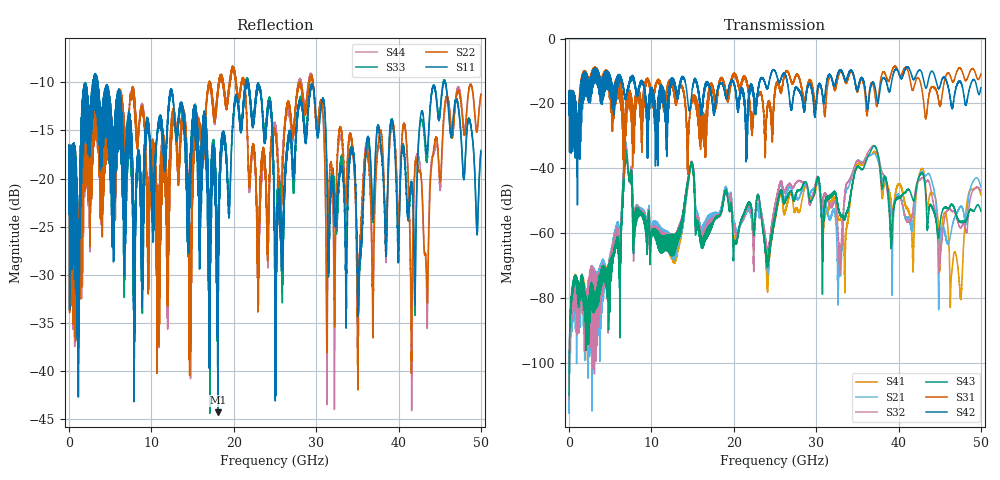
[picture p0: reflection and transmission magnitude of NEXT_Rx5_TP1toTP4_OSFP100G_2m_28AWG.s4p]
! Touchstone data
! Created: 27-Feb-2019 by IdEM 12 (12.1.0)
! COMMENTS
!  Created Wed Feb 27 12:03:36 2019
!  64 Port Network Data from SP1.SP block
!  freq  magS1_1  angS1_1  magS1_2  angS1_2  magS1_3  angS1_3  magS1_4  angS1_4
!  magS1_5  angS1_5  magS1_6  angS1_6  magS1_7  angS1_7  magS1_8  angS1_8
!  magS1_9  angS1_9  magS1_10  angS1_10  magS1_11  angS1_11  magS1_12  angS1_12
!  magS1_13  angS1_13  magS1_14  angS1_14  magS1_15  angS1_15  magS1_16  angS1_16
!  magS1_17  angS1_17  magS1_18  angS1_18  magS1_19  angS1_19  magS1_20  angS1_20
!  magS1_21  angS1_21  magS1_22  angS1_22  magS1_23  angS1_23  magS1_24  angS1_24
!  magS1_25  angS1_25  magS1_26  angS1_26  magS1_27  angS1_27  magS1_28  angS1_28
!  magS1_29  angS1_29  magS1_30  angS1_30  magS1_31  angS1_31  magS1_32  angS1_32
!  magS1_33  angS1_33  magS1_34  angS1_34  magS1_35  angS1_35  magS1_36  angS1_36
!  magS1_37  angS1_37  magS1_38  angS1_38  magS1_39  angS1_39  magS1_40  angS1_40
!  magS1_41  angS1_41  magS1_42  angS1_42  magS1_43  angS1_43  magS1_44  angS1_44
!  magS1_45  angS1_45  magS1_46  angS1_46  magS1_47  angS1_47  magS1_48  angS1_48
!  magS1_49  angS1_49  magS1_50  angS1_50  magS1_51  angS1_51  magS1_52  angS1_52
!  magS1_53  angS1_53  magS1_54  angS1_54  magS1_55  angS1_55  magS1_56  angS1_56
!  magS1_57  angS1_57  magS1_58  angS1_58  magS1_59  angS1_59  magS1_60  angS1_60
!  magS1_61  angS1_61  magS1_62  angS1_62  magS1_63  angS1_63  magS1_64  angS1_64
!  magS2_1  angS2_1  magS2_2  angS2_2  magS2_3  angS2_3  magS2_4  angS2_4
!  magS2_5  angS2_5  magS2_6  angS2_6  magS2_7  angS2_7  magS2_8  angS2_8
!  magS2_9  angS2_9  magS2_10  angS2_10  magS2_11  angS2_11  magS2_12  angS2_12
!  magS2_13  angS2_13  magS2_14  angS2_14  magS2_15  angS2_15  magS2_16  angS2_16
!  magS2_17  angS2_17  magS2_18  angS2_18  magS2_19  angS2_19  magS2_20  angS2_20
!  magS2_21  angS2_21  magS2_22  angS2_22  magS2_23  angS2_23  magS2_24  angS2_24
!  magS2_25  angS2_25  magS2_26  angS2_26  magS2_27  angS2_27  magS2_28  angS2_28
!  magS2_29  angS2_29  magS2_30  angS2_30  magS2_31  angS2_31  magS2_32  angS2_32
!  magS2_33  angS2_33  magS2_34  angS2_34  magS2_35  angS2_35  magS2_36  angS2_36
!  magS2_37  angS2_37  magS2_38  angS2_38  magS2_39  angS2_39  magS2_40  angS2_40
!  magS2_41  angS2_41  magS2_42  angS2_42  magS2_43  angS2_43  magS2_44  angS2_44
!  magS2_45  angS2_45  magS2_46  angS2_46  magS2_47  angS2_47  magS2_48  angS2_48
!  magS2_49  angS2_49  magS2_50  angS2_50  magS2_51  angS2_51  magS2_52  angS2_52
!  magS2_53  angS2_53  magS2_54  angS2_54  magS2_55  angS2_55  magS2_56  angS2_56
!  magS2_57  angS2_57  magS2_58  angS2_58  magS2_59  angS2_59  magS2_60  angS2_60
!  magS2_61  angS2_61  magS2_62  angS2_62  magS2_63  angS2_63  magS2_64  angS2_64
!  magS3_1  angS3_1  magS3_2  angS3_2  magS3_3  angS3_3  magS3_4  angS3_4
!  magS3_5  angS3_5  magS3_6  angS3_6  magS3_7  angS3_7  magS3_8  angS3_8
!  magS3_9  angS3_9  magS3_10  angS3_10  magS3_11  angS3_11  magS3_12  angS3_12
!  magS3_13  angS3_13  magS3_14  angS3_14  magS3_15  angS3_15  magS3_16  angS3_16
!  magS3_17  angS3_17  magS3_18  angS3_18  magS3_19  angS3_19  magS3_20  angS3_20
!  magS3_21  angS3_21  magS3_22  angS3_22  magS3_23  angS3_23  magS3_24  angS3_24
!  magS3_25  angS3_25  magS3_26  angS3_26  magS3_27  angS3_27  magS3_28  angS3_28
!  magS3_29  angS3_29  magS3_30  angS3_30  magS3_31  angS3_31  magS3_32  angS3_32
!  magS3_33  angS3_33  magS3_34  angS3_34  magS3_35  angS3_35  magS3_36  angS3_36
!  magS3_37  angS3_37  magS3_38  angS3_38  magS3_39  angS3_39  magS3_40  angS3_40
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# Hz S MA R 50
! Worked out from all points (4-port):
!   5000 points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, 10 MHz to 50 GHz, reference 50 ohm
!   strongest paths, dB at 10 MHz, 12.51 GHz, 25.01 GHz, 37.51 GHz, 50 GHz:
!     S42: -18.1, -13.1, -10.0, -19.7, -15.2
!     S31: -18.0, -14.0, -15.8, -18.9, -11.0
!     S43: -110.1, -65.7, -55.2, -35.7, -53.2
!     S32: -111.4, -65.8, -51.8, -35.7, -46.9
!     S21: -109.6, -66.0, -52.0, -37.7, -45.8
!     S41: -110.0, -65.8, -55.7, -37.2, -48.3
!   lowest |S11| = -44.3 dB at 18.09 GHz (marker M1), VSWR 1.01, Z = 49.5 + j0.362 ohm
!   |S11| at or under -10 dB: 3.49 GHz to 21.47 GHz (17.98 GHz wide, 144 % of centre); 21.77 GHz to 45.47 GHz (23.7 GHz wide, 70.5 % of centre); 45.66 GHz to end of sweep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
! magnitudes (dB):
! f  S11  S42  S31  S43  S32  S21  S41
! 10 MHz  -17.7  -18.1  -18.0  -110.1  -111.4  -109.6  -110.0
! 6.92 GHz  -16.6  -17.4  -20.1  -35.7  -34.7  -33.1  -34.1
! 18.09 GHz  -44.3  -14.9  -16.7  -54.7  -54.5  -54.4  -54.4
! 32.82 GHz  -19.4  -9.9  -10.6  -53.3  -66.0  -70.0  -55.8
! 37.1 GHz  -19.9  -14.5  -16.7  -33.2  -33.2  -35.5  -34.8
! 47.5 GHz  -14.7  -13.2  -9.1  -56.5  -58.3  -51.8  -79.1
! 50 GHz  -17.2  -15.2  -11.0  -53.2  -46.9  -45.8  -48.3
